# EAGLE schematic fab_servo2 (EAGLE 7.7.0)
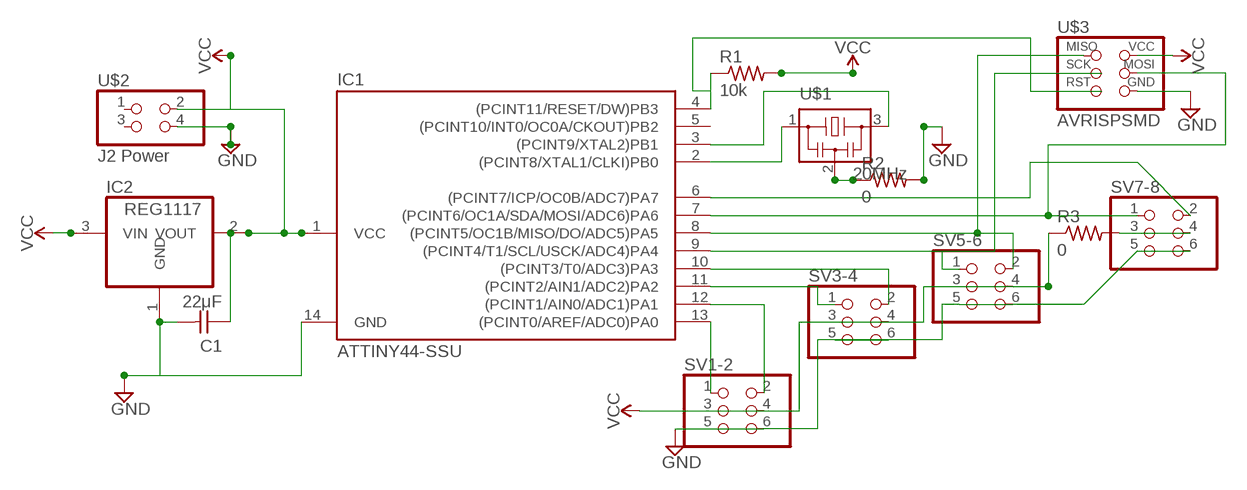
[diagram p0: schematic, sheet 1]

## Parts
C1  22μF  CAP-UNPOLARIZEDFAB  [C1206FAB]
IC1  ATTINY44-SSU  [SOIC14]
IC2  REG1117  [SOT223]
R1  10k  RES-US1206FAB  [R1206FAB]
R2  0  RES-US1206FAB  [R1206FAB]
R3  0  RES-US1206FAB  [R1206FAB]
SV1-2  PINHD-2X3-SMD  [2X03SMD]
SV3-4  PINHD-2X3-SMD  [2X03SMD]
SV5-6  PINHD-2X3-SMD  [2X03SMD]
SV7-8  PINHD-2X3-SMD  [2X03SMD]
U$1  20MHz  RESONATOR  [EFOBM]
U$2  J2 Power  PINHD-2X2-SMD  [2X02SMD]
U$3  AVRISPSMD  [2X03SMD]

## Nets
GND: C1.2 IC1.14(GND) IC2.1(GND) R2.2 SV1-2.5 SV1-2.6 SV3-4.5 SV3-4.6 SV5-6.5 SV5-6.6 SV7-8.5 SV7-8.6 U$2.4 U$3.6(GND)
N$1: IC1.7((PCINT6/OC1A/SDA/MOSI/ADC6)PA6) SV7-8.1 U$3.4(MOSI)
N$2: IC1.4((PCINT11/RESET/DW)PB3) R1.1
N$3: IC1.6((PCINT7/ICP/OC0B/ADC7)PA7) SV7-8.2
N$4: IC1.3((PCINT9/XTAL2)PB1) U$1.3
N$5: IC1.2((PCINT8/XTAL1/CLKI)PB0) U$1.1
N$6: IC1.13((PCINT0/AREF/ADC0)PA0) SV1-2.1
N$7: IC1.12((PCINT1/AIN0/ADC1)PA1) SV1-2.2
N$8: IC1.11((PCINT2/AIN1/ADC2)PA2) SV3-4.1
N$9: IC1.10((PCINT3/T0/ADC3)PA3) SV3-4.2
N$10: IC1.9((PCINT4/T1/SCL/USCK/ADC4)PA4) SV5-6.1
N$11: IC1.8((PCINT5/OC1B/MISO/DO/ADC5)PA5) SV5-6.2 U$3.1(MISO)
N$12: R2.1 U$1.2
N$13: R3.2 SV7-8.3 SV7-8.4
N$14: C1.1
VCC: IC1.1(VCC) IC2.2(VOUT) IC2.3(VIN) R1.2 R3.1 SV1-2.3 SV1-2.4 SV3-4.3 SV3-4.4 SV5-6.3 SV5-6.4 U$2.2 U$3.2(VCC)
Unconnected: IC1.5((PCINT10/INT0/OC0A/CKOUT)PB2) U$2.1 U$2.3 U$3.3(SCK) U$3.5(RST)

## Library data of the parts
C1 = fab:CAP-UNPOLARIZED
IC1 = fab:ATTINY44
IC2 = burr-brown:REG1117: 800mA and 1A Low Dropout (LDO) Positive Regulator 1.8V, 2.5V, 2.85V, 3.3V, 5V, and Adj; MPN: REG1117; OC_FARNELL: 1097566; OC_NEWARK: 14P6981
R1-R3 = fab:RES-US: Resistor (US Symbol)
SV1-2 SV3-4 SV5-6 SV7-8 = fab:PINHD-2X3-SMD: PIN HEADER
U$1 = fab:RESONATOR
U$2 = fab:PINHD-2X2-SMD
U$3 = fab:AVRISP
